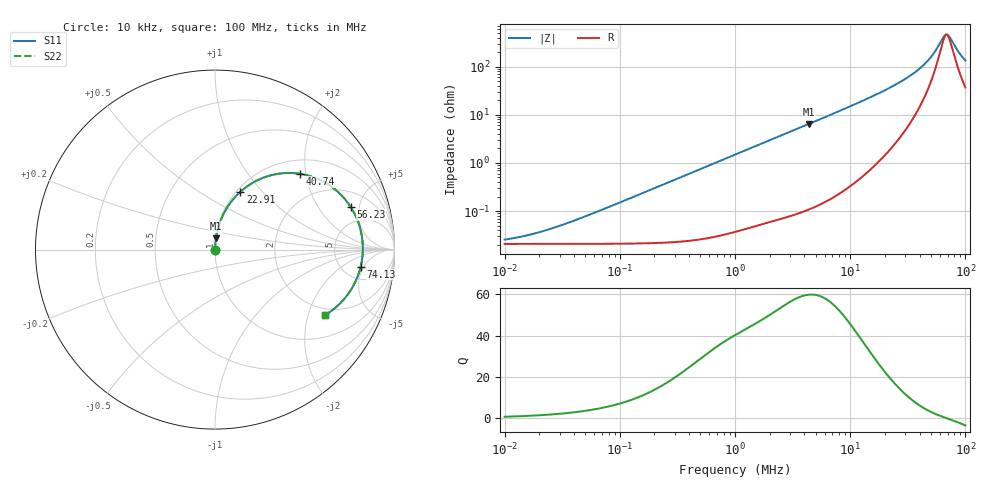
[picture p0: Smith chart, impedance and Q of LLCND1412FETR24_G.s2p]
! LLCND1412FETR24_G  S-PARAMETER MODEL  ( Standard Model )
! Model Generated by TAIYO YUDEN Corporation (http://www.ty-top.com)
! Version 1.0
! TAIYO YUDEN Control No. 231226
! Copyright(c) 2023 TAIYO YUDEN CO.,LTD. All Rights Reserved.
! Product Description (link to TY-COMPAS)
! https://ds.yuden.co.jp/TYCOMPAS/or/detail?pn=LLCND1412FETR24MG&u=M
! Products Name : Inductors
! Characteristics :
!  Inductance : 0.24 [uH] , SRF(min) : - [Hz] , DC Resistance(max) : 24 [mOhm]
!  Rated Current : Saturation  5.5 [A] (dL = 30 [%]), Temp Rise  4.3 [A] (dT = 40 [degC])
!  Case Size : 1.4 x 1.2 / 0.055 x 0.047 [mm/inch] , Thickness : 0.65 / 0.026 [mm/inch]
!  (Conditions: Temperature = 25 [degC] , DC Bias Current = 0 [A])
! External Node Assignments :
!  1  o---GGG---o  2
! GND o---------o GND
! Frequency Range : 10kHz  -  100MHz  [ 402 STEP ]
# MHz S RI R 50
! Freq[MHz].  S11 Real  S11 Imag  S21 Real  S21 Imag  S12 Real  S12 Imag  S22 Real  S22 Imag
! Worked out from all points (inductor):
!   401 points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, 10 kHz to 100 MHz, reference 50 ohm
!   read as one part in series: L = 238 nH near 42.66 kHz
!   highest Q = 59.9 at 4.365 MHz (marker M1), where L = 234 nH
!   self-resonance near 68.69 MHz
!   S11 on the Smith chart (normalised r, x): 10 kHz: 1.00, +0.00; 22.91 MHz: 1.04, +0.76; 40.74 MHz: 1.32, +1.86; 56.23 MHz: 3.22, +4.10; 74.13 MHz: 7.49, -4.27; 100 MHz: 1.74, -2.58
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0.01  0.000208 0.000149  0.9998 -0.000149  0.9998 -0.000149  0.000208 0.000149
0.013804  0.000208 0.000206  0.9998 -0.000206  0.9998 -0.000206  0.000208 0.000206
0.019953  0.000208 0.000298  0.9998 -0.000298  0.9998 -0.000298  0.000208 0.000298
0.046774  0.000209 0.000698  0.9998 -0.000698  0.9998 -0.000698  0.000209 0.000698
0.218776  0.000229 0.00326  0.9998 -0.00326  0.9998 -0.00326  0.000229 0.00326
1  0.000589 0.0148  0.9994 -0.0148  0.9994 -0.0148  0.000589 0.0148
4.365158  0.00518 0.0639  0.9948 -0.0639  0.9948 -0.0639  0.00518 0.0639
4.677351  0.00586 0.0685  0.9941 -0.0685  0.9941 -0.0685  0.00586 0.0685
12.30269  0.0381 0.1789  0.9619 -0.1789  0.9619 -0.1789  0.0381 0.1789
16.98244  0.0742 0.2446  0.9258 -0.2446  0.9258 -0.2446  0.0742 0.2446
21.87762  0.1273 0.309  0.8727 -0.309  0.8727 -0.309  0.1273 0.309
22.90868  0.1406 0.3216  0.8594 -0.3216  0.8594 -0.3216  0.1406 0.3216
30.90295  0.2696 0.4007  0.7304 -0.4007  0.7304 -0.4007  0.2696 0.4007
40.73803  0.4756 0.4219  0.5244 -0.4219  0.5244 -0.4219  0.4756 0.4219
48.97788  0.646 0.3526  0.354 -0.3526  0.354 -0.3526  0.646 0.3526
56.23413  0.7564 0.2371  0.2436 -0.2371  0.2436 -0.2371  0.7564 0.2371
66.06934  0.8217 0.049  0.1783 -0.049  0.1783 -0.049  0.8217 0.049
69.1831  0.8235 -0.00901  0.1765 0.00901  0.1765 0.00901  0.8235 -0.00901
74.13102  0.8119 -0.0946  0.1881 0.0946  0.1881 0.0946  0.8119 -0.0946
87.09636  0.727 -0.2667  0.273 0.2667  0.273 0.2667  0.727 -0.2667
95.49926  0.6535 -0.3377  0.3465 0.3377  0.3465 0.3377  0.6535 -0.3377
100  0.6133 -0.3646  0.3867 0.3646  0.3867 0.3646  0.6133 -0.3646
